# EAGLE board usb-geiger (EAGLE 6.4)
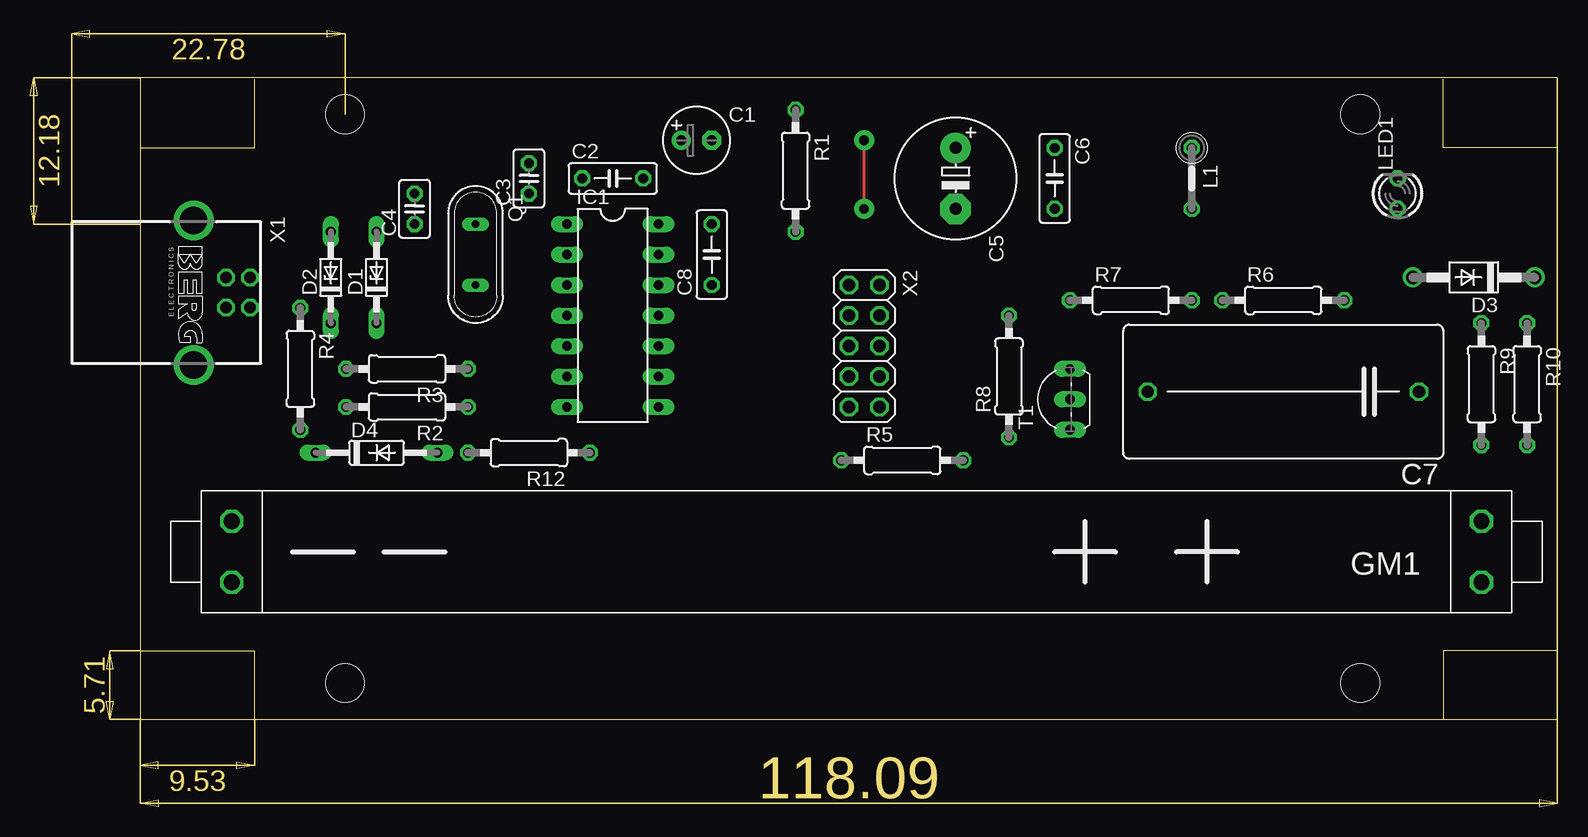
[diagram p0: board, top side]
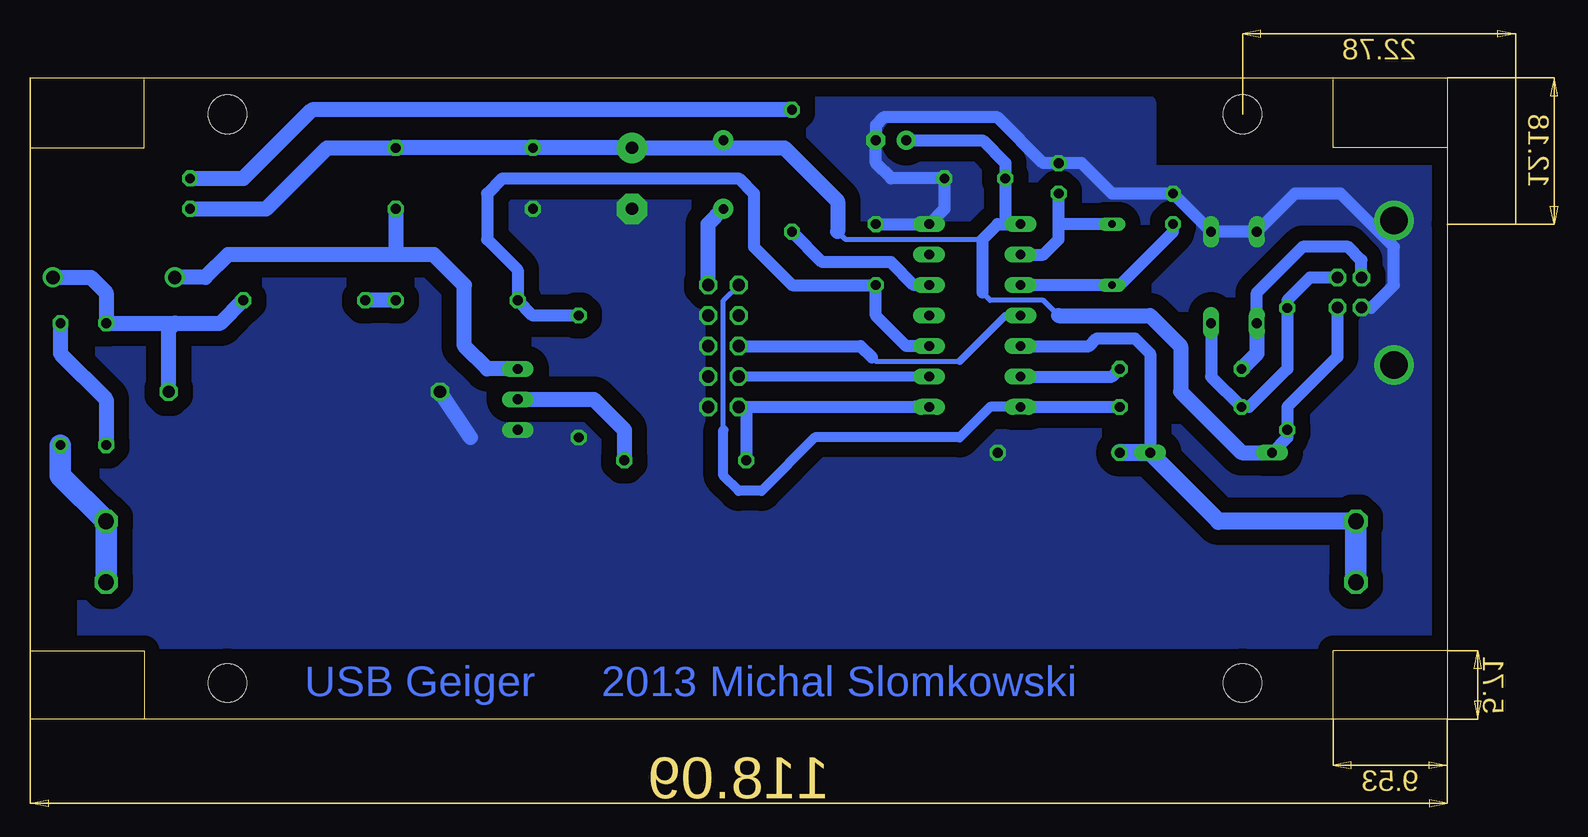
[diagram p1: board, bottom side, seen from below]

Size 127.3 x 64.73 mm. Coordinates in mm from the lower left corner, seen from the top.
Outline: 18.72,7.29 9.19,7.29 9.19,13
Outline: 18.72,7.29 117.78,7.29
Outline: 117.78,7.29 127.29,7.29 127.29,60.74 9.19,60.74 9.19,54.91
Outline: 9.19,54.91 9.19,13
Outline: 9.19,54.91 18.72,54.91 18.72,60.62
Outline: 127.3,54.91 117.78,54.91 117.78,60.62
Outline: 18.72,7.29 18.72,13 9.19,13
Outline: 127.3,13 117.78,13 117.78,7.29
Copper layers (1*16): Top 0.035mm / dielectric 1.5mm / Bottom 0.035mm
Design rules "default": minimum track width 10mil, minimum drill 24mil, track to track 8mil, track to pad 8mil, pad to pad 8mil, via to via 8mil, smd to smd 8mil, copper to edge 40mil, drill to drill 8mil, minimum pad ring 10mil, minimum via ring 8mil, stop-mask expansion 4mil, vias tented up to drill 0mil, thermal gap 10mil
Holes 3.2 mm at 110.86,57.72 26.26,57.72 26.26,10.31 110.86,10.31

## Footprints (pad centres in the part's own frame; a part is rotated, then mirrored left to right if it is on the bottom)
E2,5-6 = drill 0.813 pad 1.6: + -1.27,0 | drill 0.813 pad 1.6 octagon: - 1.27,0
C050-025X075 = drill 0.813 octagon: 1 -2.54,0; 2 2.54,0
C025-025X050 = drill 0.813 octagon: 1 -1.27,0; 2 1.27,0
E5-10,5 = drill 1.016 pad 2.54: + -2.54,0 | drill 1.016 pad 2.54 octagon: - 2.54,0
C225-113X268 = drill 1.016 octagon: 1 -11.303,0; 2 11.303,0
DO34Z7 = drill 0.813 long: A 3.81,0; C -3.81,0
DO41-10 = drill 1.118: A 5.08,0; C -5.08,0
DO35-10 = drill 0.813 long: A 5.08,0; C -5.08,0
STS-5 = drill 1.3 octagon: MINUS1 66.04,0; MINUS2 66.04,-5.08; PLUS1 -38.1,0; PLUS2 -38.1,-5.08
DIL14 = drill 0.813 long: 1 -7.62,-3.81; 2 -5.08,-3.81; 3 -2.54,-3.81; 4 0,-3.81; 5 2.54,-3.81; 6 5.08,-3.81; 7 7.62,-3.81; 8 7.62,3.81; 9 5.08,3.81; 10 2.54,3.81; 11 0,3.81; 12 -2.54,3.81; 13 -5.08,3.81; 14 -7.62,3.81
0207/5V = drill 0.813 octagon: 1 -2.54,0; 2 2.54,0
LED3MM = drill 0.813 octagon: A -1.27,0; K 1.27,0
QS = drill 0.61 long: 1 -2.54,0; 2 2.54,0
0207/10 = drill 0.813 octagon: 1 -5.08,0; 2 5.08,0
TO92-EBC = drill 0.813 long: B 0,-1.27; C 2.54,-1.27; E -2.54,-1.27
PN61729-S = drill 0.95 octagon: 1 1.25,4.71; 2 -1.25,4.71; 3 -1.25,2.71; 4 1.25,2.71 | drill 2.3 pad 2.9: S1 -6.02,0; S2 6.02,0
2X05 = drill 1.016 octagon: 1 -5.08,-1.27; 2 -5.08,1.27; 3 -2.54,-1.27; 4 -2.54,1.27; 5 0,-1.27; 6 0,1.27; 7 2.54,-1.27; 8 2.54,1.27; 9 5.08,-1.27; 10 5.08,1.27

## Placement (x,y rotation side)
C1  47u  [E2,5-6]  55.55,55.55 0 top
C2  100n  [C050-025X075]  48.56,52.37 0 top
C3  22p  [C025-025X050]  41.58,52.37 90 top
C4  22p  [C025-025X050]  32.05,49.83 90 top
C5  220u  [E5-10,5]  77.14,52.37 270 top
C6  100n  [C050-025X075]  85.39,52.37 270 top
C7  100n/600V  [C225-113X268]  104.44,34.59 180 top
C8  10n  [C050-025X075]  56.81,46.02 90 top
D1  3V6  [DO34Z7]  28.88,44.12 90 top
D2  3V6  [DO34Z7]  25.07,44.12 90 top
D3  1N4937  [DO41-10]  120.32,44.12 180 top
D4  BAT42  [DO35-10]  28.88,29.51 0 top
GM1  STS-5  [STS-5]  82.85,18.71 180 top
IC1  TINY24  [DIL14]  48.56,40.94 270 top
L1  10m  [0207/5V]  96.82,52.37 270 top
LED1  [LED3MM]  113.97,51.1 90 top
Q1  16MHz  [QS]  37.13,46.02 270 top
R1  2k2  [0207/10]  63.8,53.01 270 top
R2  68  [0207/10]  31.41,33.32 180 top
R3  68  [0207/10]  31.41,36.49 180 top
R4  1k5  [0207/10]  22.53,36.49 270 top
R5  1k  [0207/10]  72.69,28.88 0 top
R6  1M  [0207/10]  104.44,42.21 0 top
R7  1M  [0207/10]  91.74,42.21 0 top
R8  4k7  [0207/10]  81.58,35.86 90 top
R9  1M  [0207/10]  120.95,35.23 270 top
R10  4M7  [0207/10]  124.76,35.23 270 top
R12  330k  [0207/10]  41.58,29.51 180 top
T1  MPSA44  [TO92-EBC]  85.39,33.95 90 top
X1  PN61729-S  [PN61729-S]  13.64,42.84 270 top
X2  [2X05]  69.52,38.4 270 top

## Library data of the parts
C1-C8 L1 R1-R10 R12 = rcl
D1-D4 = diode
GM1 T1 = geiger
IC1 = avr-7
LED1 = led
Q1 = special
X1 = con-berg; OC_FARNELL: unknown; OC_NEWARK: unknown
X2 = pinhead

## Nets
+5V: C1.+ C2.1 C5.+ C6.1 D4.C IC1.1 L1.1 LED1.A R4.2 X1.1 X2.2
GND: C1.- C2.2 C3.2 C4.2 C5.- C6.2 C7.2 C8.2 D1.A D2.A IC1.14 R8.1 R12.1 T1.E X1.4 X1.S1 X1.S2 X2.4 X2.6 X2.8 X2.10
N$1: R6.1 R7.2
N$2: D3.A L1.2 T1.C
N$3: R5.2 T1.B
N$4: C7.1 D3.C R6.2 R9.1
N$5: R9.2 R10.1
N$6: GM1.PLUS1 GM1.PLUS2 R10.2
N$7: C8.1 IC1.10 R7.1 R8.2
N$8: IC1.6 R3.1
N$9: D4.A GM1.MINUS1 GM1.MINUS2 IC1.5 R12.2
N$10: IC1.8 R5.1 X2.9
N$12: IC1.7 R2.1 X2.1
N$13: IC1.4 X2.5
N$15: IC1.9 X2.7
N$16: D1.C R2.2 R4.1 X1.2
N$17: D2.C R3.2 X1.3
N$18: C4.1 IC1.3 Q1.2
N$19: C3.1 IC1.2 Q1.1
N$20: IC1.12 R1.2
N$21: LED1.K R1.1

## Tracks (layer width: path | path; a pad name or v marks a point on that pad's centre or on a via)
+5V  (via drill 0.8 pad 1.68)
  Top 0.254: v69.52,49.83 v69.52,55.55
  Bottom 0.406: 41.58,40.94 42.84,42.21 47.29,42.21 47.92,42.84 | 47.92,47.29 59.35,47.29 59.99,47.92
  Bottom 1.016: 47.92,42.84 47.92,47.29 46.66,48.56 46.02,48.56 | 46.02,48.56 IC1.1 | 46.02,48.56 C2.1 46.02,53.64 47.92,55.55 C1.+ | D4.C 22.53,30.78 R4.2 22.53,33.32 18.34,37.5 X1.1
  Bottom 1.27: X2.2 70.78,48.56 v69.52,49.83 | v69.52,55.55 70.15,54.91 | 70.15,54.91 64.44,54.91 59.99,50.47 59.99,47.92 | 70.15,54.91 C5.+ C6.1 L1.1 102.54,54.91 107.62,49.83 LED1.A | 41.58,40.94 33.95,40.94 31.41,38.4 31.41,34.59 26.34,29.51 D4.C
GND
  Bottom 1.016: C8.2 IC1.14 51.1,49.83 C2.2 55.55,52.37 56.81,53.64 C1.- 56.81,56.81 56.18,57.45 46.66,57.45 42.84,53.64 C3.2 39.67,53.64 37.13,51.1 C4.2 D1.A D2.A 21.89,51.1 18.08,51.1 13.64,46.66 13.64,43.48 15.54,41.58 16.33,41.58 X1.4
  Bottom 1.27: 90.6,30.78 C7.2
  pour Bottom (isolate 1.27, no thermals): 122.86,13.63 122.86,58.72 33.95,58.72 33.95,53.01 9.83,53.01 9.83,13.63
N$1
  Bottom 1.27: R7.2 R6.1
N$2
  Bottom 1.27: L1.2 96.82,46.02 | 96.82,46.02 110.79,46.02 112.7,44.12 D3.A | 96.82,46.02 93.65,46.02 91.11,43.48 91.11,38.4 89.2,36.49 T1.C
N$3
  Bottom 1.27: T1.B 80.31,33.95 77.77,31.41 R5.2
N$4
  Bottom 1.27: D3.C 122.22,44.12 120.95,42.84 R9.1 115.24,40.3 | 115.24,40.3 111.43,40.3 R6.2 | C7.1 115.74,39.8 115.24,40.3
N$5
  Bottom 1.27: R10.1 124.76,37.77 120.95,33.95 R9.2
N$6
  Bottom 1.778: R10.2 124.76,27.61 GM1.PLUS2 GM1.PLUS1
N$7
  Bottom 1.016: R8.2 85.39,40.94 R7.1 86.66,44.75 89.2,47.29 89.2,51.1 87.93,52.37 68.25,52.37 66.98,51.1 66.98,46.66 63.8,43.48 C8.1 56.81,40.94 54.27,38.4 IC1.10
N$8
  Bottom 1.016: IC1.6 37.13,35.86 R3.1
N$9
  Bottom 1.016: IC1.5 39.04,38.4 38.4,39.04 35.23,39.04 33.95,37.77 D4.A
  Bottom 1.422: GM1.MINUS2 28.24,23.8 D4.A R12.2
  Bottom 1.778: GM1.MINUS1 GM1.MINUS2
N$10
  Bottom 1.016: 53.64,33.32 IC1.8 67.61,33.32 | 67.61,33.32 R5.1 | X2.9 67.61,33.32
N$12
  Bottom 0.406: 69.52,31.41 69.52,42.21 X2.1
  Bottom 0.813: IC1.7 47.29,33.32 49.83,30.78 61.9,30.78 66.34,26.34 68.25,26.34 69.52,27.61 69.52,31.41
  Bottom 1.016: IC1.7 R2.1
N$13
  Bottom 0.406: 49.83,37.13 56.81,37.13 57.13,37.45
  Bottom 0.61: 49.83,37.13 46.02,40.94 IC1.4
  Bottom 1.016: X2.5 58.09,38.4 57.13,37.45
N$15
  Bottom 0.813: IC1.9 X2.7
N$16
  Bottom 1.016: D1.C 28.88,35.86 R2.2 25.7,33.32 22.53,36.49 R4.1 22.53,42.21 20.64,44.09 X1.2
N$17
  Bottom 1.016: X1.3 16.35,45.55 17.45,46.66 21.26,46.66 25.07,42.84 D2.C
  Bottom 1.27: D2.C 25.07,37.77 R3.2
N$18
  Bottom 1.016: IC1.3 Q1.2 36.5,43.48 32.05,47.92 C4.1
N$19
  Bottom 1.016: Q1.1 41.58,48.56 | 41.58,48.56 C3.1 | IC1.2 42.84,46.02 41.58,47.29 41.58,48.56
N$20
  Bottom 1.016: IC1.12 53.64,43.48 55.55,45.38 61.26,45.38 R1.2
N$21
  Bottom 1.27: R1.1 103.81,58.09 109.52,52.37 LED1.K
N$22  (via drill 1)
  other vias: 26.26,57.72
N$25  (via drill 1)
  other vias: 26.26,10.31
N$26  (via drill 1)
  other vias: 110.86,57.72
N$27  (via drill 1)
  other vias: 110.86,10.31

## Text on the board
Bottom: 2013 Michal Slomkowski | USB Geiger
